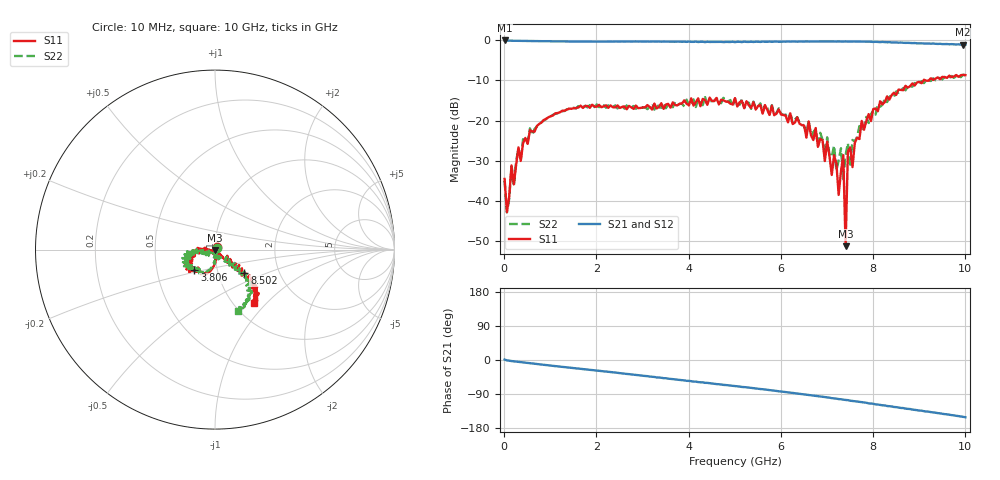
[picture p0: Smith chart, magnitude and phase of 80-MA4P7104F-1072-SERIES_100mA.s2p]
!Agilent Technologies,E8364C,MY48140145,A.09.42.15
!Agilent E8364C: A.09.42.15
!Date: Wednesday, December 02, 2020 07:36:07
!Correction: S11(Full 2 Port(1,2))
!S21(Full 2 Port(1,2))
!S12(Full 2 Port(1,2))
!S22(Full 2 Port(1,2))
!S2P File: Measurements: S11, S21, S12, S22:
# Hz S  dB  R 50
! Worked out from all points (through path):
!   201 points, 10 MHz to 10 GHz, reference 50 ohm
!   highest |S21| = -0.06 dB at 10 MHz (marker M1); lowest = -1.1 dB at 9.95 GHz (marker M2)
!   group delay of S21, straight-line fit = 41 ps
!   lowest |S11| = -51.2 dB at 7.403 GHz (marker M3), VSWR 1.01, Z = 50 - j0.274 ohm
!   |S11| at or under -10 dB: start of sweep to 9.091 GHz; 9.138 GHz to 9.208 GHz (69.85 MHz wide, 0.762 % of centre)
!   |S22| runs from -42.8 to -8.6 dB; largest |S21 - S12| = 0.022
!   S11 on the Smith chart (normalised r, x): 10 MHz: 1.02, +0.03; 3.806 GHz: 0.78, -0.18; 8.502 GHz: 1.33, -0.36; 10 GHz: 1.23, -0.85
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1e7  -34.51 57.6  -0.06 1.2  -0.07 -0.1  -35.01 40.8
5.995e7  -42.78 -50.7  -0.11 -1.0  -0.11 -1.1  -42.83 -64.0
1.5985e8  -31.16 -76.4  -0.13 -2.8  -0.13 -2.8  -31.30 -74.8
2.098e8  -35.86 -68.0  -0.13 -3.5  -0.14 -3.5  -36.34 -78.7
5.5945e8  -22.38 -92.0  -0.21 -8.6  -0.20 -8.6  -21.95 -91.6
1.7083e9  -16.86 -114.9  -0.34 -24.1  -0.32 -23.9  -16.61 -120.4
3.35665e9  -16.60 -135.3  -0.32 -46.2  -0.33 -46.4  -16.71 -129.1
3.8062e9  -15.81 -135.0  -0.37 -52.6  -0.35 -52.6  -15.86 -136.9
5.005e9  -14.43 -152.6  -0.49 -69.0  -0.45 -68.8  -14.48 -165.6
6.7033e9  -24.83 177.6  -0.30 -94.2  -0.27 -93.8  -22.90 176.3
7.15285e9  -28.62 179.7  -0.33 -101.3  -0.33 -101.6  -26.20 -134.1
7.25275e9  -38.49 -176.6  -0.29 -103.1  -0.30 -102.8  -29.83 -155.1
7.35265e9  -28.61 -59.9  -0.33 -104.7  -0.29 -104.3  -34.53 -61.9
7.4026e9  -51.24 -92.9  -0.31 -105.5  -0.31 -105.5  -28.57 -106.0
7.45255e9  -27.74 -71.3  -0.33 -105.9  -0.32 -106.4  -25.62 -60.6
7.5025e9  -26.65 -42.6  -0.33 -107.4  -0.29 -106.9  -31.59 -48.8
7.55245e9  -31.57 -45.7  -0.32 -108.0  -0.34 -108.2  -24.82 -71.6
7.7023e9  -24.58 -46.0  -0.35 -110.5  -0.38 -110.9  -21.35 -50.9
8.35165e9  -14.79 -34.7  -0.49 -122.0  -0.52 -122.0  -14.11 -45.8
8.5015e9  -13.61 -38.5  -0.55 -124.4  -0.58 -124.8  -12.72 -44.6
9.95005e9  -8.62 -50.9  -1.11 -150.2  -1.12 -150.0  -8.60 -69.8
1e10  -8.68 -53.8  -1.10 -151.1  -1.09 -151.0  -8.79 -69.5
